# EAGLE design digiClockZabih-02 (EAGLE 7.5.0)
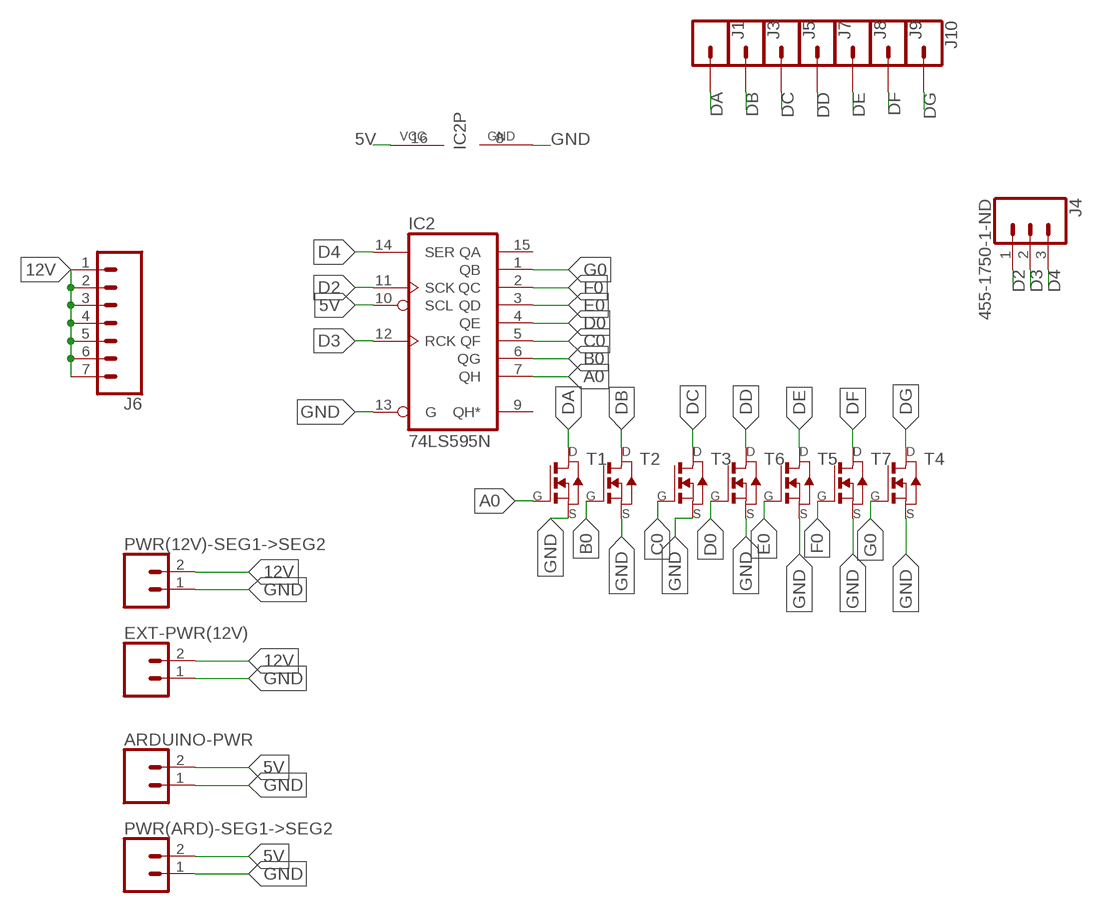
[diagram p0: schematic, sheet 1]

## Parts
ARDUINO-PWR  CONN_02  [1X02]
EXT-PWR(12V)  CONN_02PTH4  [1X02_XTRA_BIG]
IC2  74LS595N  [DIL16]
J1  CONN_01  [1X01]
J3  CONN_01  [1X01]
J4  455-1750-1-ND  CONN_03  [1X03]
J5  CONN_01  [1X01]
J6  CONN_07  [1X07]
J7  CONN_01  [1X01]
J8  CONN_01  [1X01]
J9  CONN_01  [1X01]
J10  CONN_01  [1X01]
PWR(12V)-SEG1->SEG2  CONN_02PTH4  [1X02_XTRA_BIG]
PWR(ARD)-SEG1->SEG2  CONN_02  [1X02]
T1  NMOSFETSOT23  [SOT-23]
T2  NMOSFETSOT23  [SOT-23]
T3  NMOSFETSOT23  [SOT-23]
T4  NMOSFETSOT23  [SOT-23]
T5  NMOSFETSOT23  [SOT-23]
T6  NMOSFETSOT23  [SOT-23]
T7  NMOSFETSOT23  [SOT-23]

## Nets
5V: ARDUINO-PWR.2 IC2.10(SCL) IC2.16(VCC) PWR(ARD)-SEG1->SEG2.2
12V: EXT-PWR(12V).2 J6.1 J6.2 J6.3 J6.4 J6.5 J6.6 J6.7 PWR(12V)-SEG1->SEG2.2
A0: IC2.7(QH) T1.3(G)
B0: IC2.6(QG) T2.3(G)
C0: IC2.5(QF) T3.3(G)
D0: IC2.4(QE) T6.3(G)
D2: IC2.11(SCK) J4.1
D3: IC2.12(RCK) J4.2
D4: IC2.14(SER) J4.3
DA: J1.1 T1.1(D)
DB: J3.1 T2.1(D)
DC: J5.1 T3.1(D)
DD: J7.1 T6.1(D)
DE: J8.1 T5.1(D)
DF: J9.1 T7.1(D)
DG: J10.1 T4.1(D)
E0: IC2.3(QD) T5.3(G)
F0: IC2.2(QC) T7.3(G)
G0: IC2.1(QB) T4.3(G)
GND: ARDUINO-PWR.1 EXT-PWR(12V).1 IC2.8(GND) IC2.13(G) PWR(12V)-SEG1->SEG2.1 PWR(ARD)-SEG1->SEG2.1 T1.2(S) T2.2(S) T3.2(S) T4.2(S) T5.2(S) T6.2(S) T7.2(S)
Unconnected: IC2.9(QH*) IC2.15(QA)

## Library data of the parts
ARDUINO-PWR EXT-PWR(12V) PWR(12V)-SEG1->SEG2 PWR(ARD)-SEG1->SEG2 = SparkFun-Connectors:CONN_02: Multi connection point. Often used as Generic Header-pin footprint for 0.1 inch spaced/style header connections
IC2 = 74xx-us:74*595: 8-bit SHIFT REGISTER, output latch
J1 J3 J5 J7-J10 = SparkFun-Connectors:CONN_01: Single connection point. Often used as Generic Header-pin footprint for 0.1 inch spaced/style header connections
J4 = SparkFun-Connectors:CONN_03: Multi connection point. Often used as Generic Header-pin footprint for 0.1 inch spaced/style header connections On any of the 0.1 inch spaced packages, you can populate with these: Break Away Headers - Straight (PRT-00116) Break Away Male Headers - Right Angle (PRT-00553) Female Headers (PRT-00115)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; PROD_ID: XXX-00000
J6 = SparkFun-Connectors:CONN_07: Multi connection point. Often used as Generic Header-pin footprint for 0.1 inch spaced/style header connections On any of the 0.1 inch spaced packages, you can populate with these: Break Away Headers - Straight (PRT-00116) Break Away Male Headers - Right Angle (PRT-00553) Female Headers (PRT-00115)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
T1-T7 = fab:NMOSFET: MOS FET

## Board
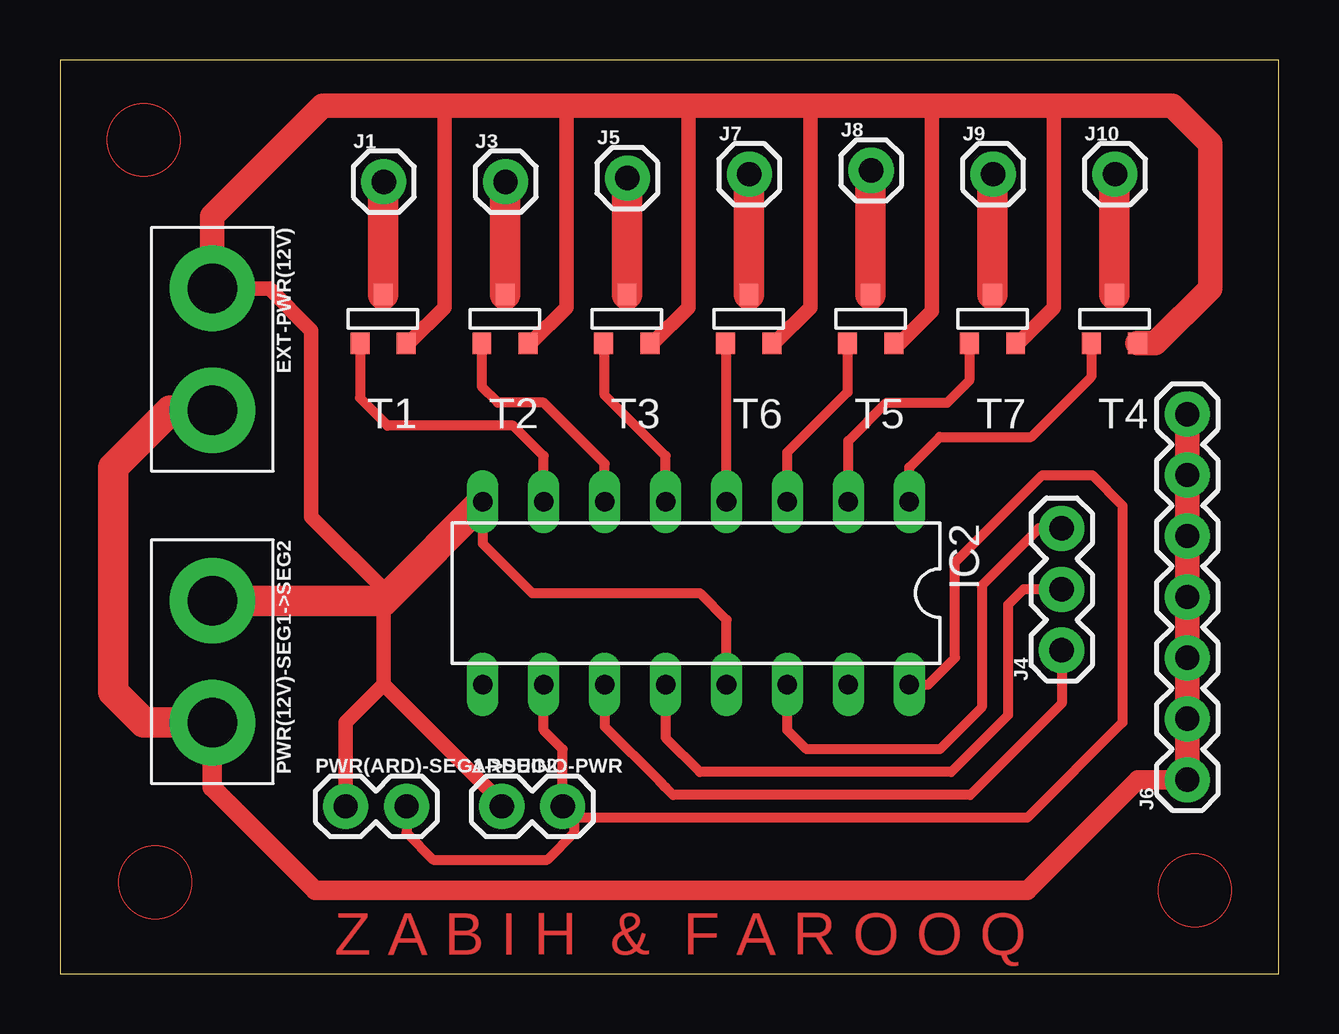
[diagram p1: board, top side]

Size 50.8 x 38.1 mm. Coordinates in mm from the lower left corner, seen from the top.
Outline: 0,0 50.8,0 50.8,38.1 0,38.1 0,0
Copper layers (1*16): Top 0.035mm / dielectric 1.5mm / Bottom 0.035mm
Design rules "default": minimum track width 10mil, minimum drill 24mil, track to track 8mil, track to pad 8mil, pad to pad 8mil, via to via 8mil, smd to smd 8mil, copper to edge 40mil, drill to drill 8mil, minimum pad ring 10mil, minimum via ring 8mil, stop-mask expansion 4mil, vias tented up to drill 0mil, thermal gap 10mil

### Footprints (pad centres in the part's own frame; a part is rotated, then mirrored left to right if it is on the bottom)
1X02 = drill 1.016 pad 1.88: 1 0,0; 2 2.54,0
1X02_XTRA_BIG = drill 2.057 pad 3.556: 1 -2.54,0; 2 2.54,0
DIL16 = drill 0.813 long: 1 -8.89,-3.81; 2 -6.35,-3.81; 3 -3.81,-3.81; 4 -1.27,-3.81; 5 1.27,-3.81; 6 3.81,-3.81; 7 6.35,-3.81; 8 8.89,-3.81; 9 8.89,3.81; 10 6.35,3.81; 11 3.81,3.81; 12 1.27,3.81; 13 -1.27,3.81; 14 -3.81,3.81; 15 -6.35,3.81; 16 -8.89,3.81
1X01 = drill 1.016 pad 1.88: 1 0,0
1X03 = drill 1.016 pad 1.88: 1 0,0; 2 2.54,0; 3 5.08,0
1X07 = drill 1.016 pad 1.88: 1 0,0; 2 2.54,0; 3 5.08,0; 4 7.62,0; 5 10.16,0; 6 12.7,0; 7 15.24,0
SOT-23 = smd 0.787 x 0.889: 1 0.025,-1.016; 2 -0.94,1.016; 3 0.991,1.016

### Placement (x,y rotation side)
ARDUINO-PWR  18.41,6.99 0 top
EXT-PWR(12V)  6.35,26.04 270 top
IC2  26.51,15.88 180 top
J1  13.49,33.02 0 top
J3  18.57,33.02 0 top
J4  41.75,13.49 90 top
J5  23.65,33.18 0 top
J6  46.99,8.1 90 top
J7  28.73,33.34 0 top
J8  33.81,33.5 0 top
J9  38.89,33.34 0 top
J10  43.97,33.34 0 top
PWR(12V)-SEG1->SEG2  6.35,13.02 270 top
PWR(ARD)-SEG1->SEG2  11.91,6.99 0 top
T1  13.49,27.3 180 top
T2  18.57,27.3 180 top
T3  23.65,27.3 180 top
T4  43.97,27.3 180 top
T5  33.81,27.3 180 top
T6  28.73,27.3 180 top
T7  38.89,27.3 180 top

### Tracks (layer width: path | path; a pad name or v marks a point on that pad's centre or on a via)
5V
  Top 0.406: IC2.10 20.16,10.16 20.95,9.37 ARDUINO-PWR.2 21.43,6.51 | IC2.16 36.2,12.06 37.31,13.18 37.31,17.14 40.96,20.8 43.02,20.8 44.29,19.53 44.29,10.48 40.32,6.51 21.43,6.51 | PWR(ARD)-SEG1->SEG2.2 14.45,5.87 15.56,4.76 20.32,4.76 21.43,5.87 21.43,6.51
12V
  Top 0.813: J6.1 44.93,8.1 40.32,3.49 10.64,3.49 6.35,7.78 PWR(12V)-SEG1->SEG2.2
  Top 1.016: J6.7 J6.6 J6.5 J6.4 J6.3 J6.2 J6.1
  Top 1.27: EXT-PWR(12V).2 4.6,23.5 2.22,21.11 2.22,11.75 3.49,10.48 PWR(12V)-SEG1->SEG2.2
A0
  Top 0.406: IC2.7 20.16,21.59 18.89,22.86 13.65,22.86 12.5,24.01 T1.3
B0
  Top 0.406: IC2.6 22.7,21.27 20.16,23.81 18.26,23.81 17.58,24.49 T2.3
C0
  Top 0.406: IC2.5 25.24,21.59 22.7,24.13 22.7,26.25 T3.3
D0
  Top 0.406: IC2.4 27.78,26.25 T6.3
D2
  Top 0.406: IC2.11 22.7,10.32 25,8.02 25.24,7.78 25.56,7.46 37.94,7.46 41.75,11.27 J4.1
D3
  Top 0.406: IC2.12 25.24,9.84 26.67,8.41 37.15,8.41 39.53,10.79 39.53,15.4 40.16,16.03 J4.2
D4
  Top 0.406: J4.3 40.8,18.57 38.42,16.19 38.42,11.11 36.67,9.37 31.11,9.37 30.32,10.16 IC2.14
DA
  Top 1.27: T1.1 13.47,32.99 J1.1
DB
  Top 1.27: T2.1 18.55,32.99 J3.1
DC
  Top 1.27: T3.1 23.63,33.15 J5.1
DD
  Top 1.27: T6.1 28.71,33.31 J7.1
DE
  Top 1.27: T5.1 33.79,33.47 J8.1
DF
  Top 1.27: T7.1 38.87,33.31 J9.1
DG
  Top 1.27: T4.1 43.95,33.31 J10.1
E0
  Top 0.406: IC2.3 30.32,21.75 32.82,24.25 T5.3
F0
  Top 0.406: IC2.2 32.86,22.23 34.45,23.81 36.99,23.81 37.9,24.73 T7.3
G0
  Top 0.406: IC2.1 35.4,21.11 36.67,22.38 40.48,22.38 42.98,24.89 T4.3
GND
  Top 0.406: IC2.13 27.78,14.76 26.67,15.88 19.68,15.88 17.62,17.94 IC2.8 14.76,16.83
  Top 0.61: T2.2 19.62,26.29 21.11,27.78 21.11,36.2 | T1.2 14.54,26.29 16.03,27.78 16.03,36.2 | T3.2 24.7,26.29 26.19,27.78 26.19,36.04 26.04,36.2 | T6.2 29.78,26.29 31.27,27.78 31.27,35.88 31.59,36.2 | T5.2 35.02,26.29 36.35,27.62 36.35,35.88 36.04,36.2 | T7.2 39.94,26.29 41.43,27.78 41.43,36.2 | ARDUINO-PWR.1 18.41,7.14 13.49,12.06 | 13.49,15.56 13.49,12.06 | PWR(ARD)-SEG1->SEG2.1 11.91,10.48 13.49,12.06 | EXT-PWR(12V).1 8.73,28.57 10.48,26.83 10.48,19.05 13.73,15.8
  Top 1.016: T4.2 45.66,26.29 47.94,28.57 47.94,34.61 46.35,36.2 41.43,36.2 36.04,36.2 31.59,36.2 26.04,36.2 21.11,36.2 16.03,36.2 10.95,36.2 6.35,31.59 EXT-PWR(12V).1
  Top 1.27: PWR(12V)-SEG1->SEG2.1 13.49,15.56 13.73,15.8 IC2.8
(copper drawn outside any net)
  shapes: Top circle x3

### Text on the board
Top: Z A B I H & F A R O O Q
